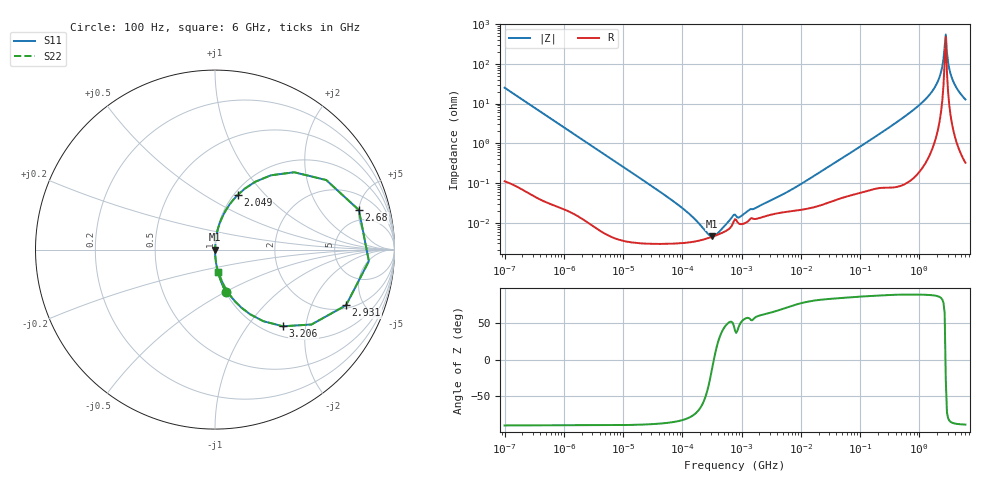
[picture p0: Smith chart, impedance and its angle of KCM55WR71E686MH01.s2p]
!Murata Part Number: KCM55WR71E686MH01
!These Parameters are Measured in Series Mode Connection
!Data Generated on Mar 13, 2026
!  o--ll--o
!Port1  Port2
!  o------o
!Operation Temp=25[degC], DC Bias Voltage=0[V]
!Freq. Start=100[Hz] Stop=6[GHz] 401[Steps]
# Hz S RI R 50
!Freq.(Hz) S11(Real) S11(Imag) S21(Real) S21(Imag) S12(Real) S12(Imag) S22(Real) S22(Imag)
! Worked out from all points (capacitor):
!   401 points, 100 Hz to 6 GHz, reference 50 ohm
!   read as one part in series: C = 63.2 uF near 109 Hz
!   lowest |Z| = 4.52 mohm at 316.4 kHz (marker M1)
!   series resonance near 340.4 kHz, so ESL is about 3.5 nH
!   S11 on the Smith chart (normalised r, x): 100 Hz: 1.00, -0.50; 2.049 GHz: 1.04, +0.71; 2.68 GHz: 3.51, +5.01; 2.931 GHz: 2.19, -3.67; 3.206 GHz: 1.18, -1.50; 6 GHz: 1.01, -0.25
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100  0.0604 -0.2359  0.9396 0.2359  0.9396 0.2359  0.0604 -0.2359
350  0.00558 -0.0716  0.9944 0.0716  0.9944 0.0716  0.00558 -0.0716
2008  0.000288 -0.0127  0.9997 0.0127  0.9997 0.0127  0.000288 -0.0127
40335  2.97e-05 -0.000625  1 0.000625  1 0.000625  2.97e-05 -0.000625
184852  3.5e-05 -9.47e-05  1 9.47e-05  1 9.47e-05  3.5e-05 -9.47e-05
316350  4.4e-05 -1.02e-05  1 1.02e-05  1 1.02e-05  4.4e-05 -1.02e-05
541393  6.17e-05 6.54e-05  0.9999 -6.54e-05  0.9999 -6.54e-05  6.17e-05 6.54e-05
774597  0.000123 0.000102  0.9999 -0.000102  0.9999 -0.000102  0.000123 0.000102
968953  9.2e-05 0.000112  0.9999 -0.000112  0.9999 -0.000112  9.2e-05 0.000112
1.555665e7  0.000241 0.00139  0.9998 -0.00139  0.9998 -0.00139  0.000241 0.00139
3.124326e8  0.0014 0.0252  0.9986 -0.0252  0.9986 -0.0252  0.0014 0.0252
1.144649e9  0.0144 0.1083  0.9856 -0.1083  0.9856 -0.1083  0.0144 0.1083
1.637704e9  0.0446 0.19  0.9554 -0.19  0.9554 -0.19  0.0446 0.19
2.048624e9  0.1274 0.3054  0.8726 -0.3054  0.8726 -0.3054  0.1274 0.3054
2.240541e9  0.2249 0.3783  0.7751 -0.3783  0.7751 -0.3783  0.2249 0.3783
2.450438e9  0.4415 0.4309  0.5585 -0.4309  0.5585 -0.4309  0.4415 0.4309
2.679998e9  0.8016 0.2204  0.1984 -0.2204  0.1984 -0.2204  0.8016 0.2204
2.931063e9  0.7299 -0.3104  0.2701 0.3104  0.2701 0.3104  0.7299 -0.3104
3.205649e9  0.3784 -0.4273  0.6216 0.4273  0.6216 0.4273  0.3784 -0.4273
3.505958e9  0.1956 -0.3603  0.8044 0.3603  0.8044 0.3603  0.1956 -0.3603
3.8344e9  0.1128 -0.2898  0.8872 0.2898  0.8872 0.2898  0.1128 -0.2898
6e9  0.0189 -0.124  0.9811 0.124  0.9811 0.124  0.0189 -0.124
